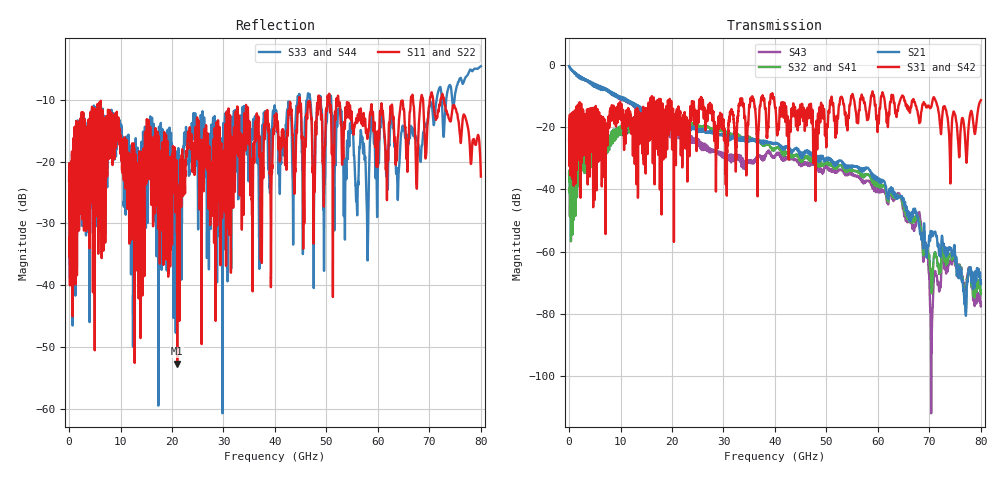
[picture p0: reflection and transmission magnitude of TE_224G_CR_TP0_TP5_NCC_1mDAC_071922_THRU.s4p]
!! Reference: tracy_3df_01a_2207
!! CHANNEL DESCRIPTION: TP0_TP5 CR Channel using 1meter DAC, CABLED NCC Host
!! MODEL DESCRIPTION: s4p, THRU
!! CONNECTOR DESCRIPTION: OSFP 200G OTB, NCC Socket
!! CABLE DESCRIPTION: 1meter 26AWG Cable
!! MODEL STATUS: Developmental
!! PORT DEFINITIONS:
!! Port  1  ----->  Side A  Side B  <-----  Port  2
!! Port  3  ----->  Side A  Side B  <-----  Port  4
# GHz S MA R 50
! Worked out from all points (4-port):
!   8000 points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, 10 MHz to 80 GHz, reference 50 ohm
!   strongest paths, dB at 10 MHz, 20.01 GHz, 40.01 GHz, 60.01 GHz, 80 GHz:
!     S31: -24.5, -26.1, -13.7, -17.6, -11.4
!     S42: -24.5, -26.1, -13.7, -17.6, -11.4
!     S21: -0.5, -19.4, -25.4, -37.4, -70.3
!     S32: -34.9, -17.8, -27.0, -39.1, -73.5
!     S41: -34.9, -17.8, -27.0, -39.1, -73.5
!     S43: -0.5, -21.7, -29.5, -41.0, -77.4
!   lowest |S11| = -52.7 dB at 21.01 GHz (marker M1), VSWR 1.00, Z = 50 + j0.231 ohm
!   |S11| at or under -10 dB: start of sweep to 44.68 GHz; 52.32 GHz to 66.38 GHz (14.06 GHz wide, 23.7 % of centre); 72.83 GHz to end of sweep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
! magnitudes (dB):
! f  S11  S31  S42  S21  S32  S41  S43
! 10 MHz  -23.1  -24.5  -24.5  -0.5  -34.9  -34.9  -0.5
! 21.01 GHz  -52.7  -17.3  -17.3  -19.9  -18.1  -18.1  -22.3
! 64.11 GHz  -13.0  -12.7  -12.7  -42.4  -42.0  -42.0  -41.4
! 68.04 GHz  -12.8  -18.8  -18.8  -52.0  -49.7  -49.7  -47.3
! 70.39 GHz  -8.8  -13.4  -13.4  -55.2  -71.8  -71.8  -94.0
! 74.58 GHz  -10.9  -15.8  -15.8  -60.3  -61.3  -61.3  -62.4
! 80 GHz  -22.4  -11.4  -11.4  -70.3  -73.5  -73.5  -77.4
